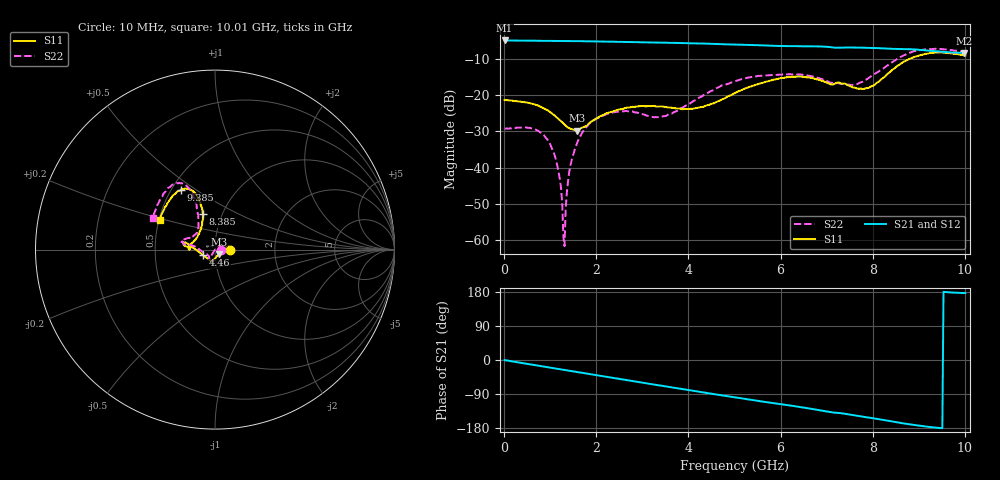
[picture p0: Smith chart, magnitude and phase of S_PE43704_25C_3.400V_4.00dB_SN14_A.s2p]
! Device ID: PE43704
! Dir: z:\PE43704\PE43704_Char_1_20130516\PE43704\AMB\3p400V\4p00dB
! Serial: 14
! Insertion: A
! Impedance: 50 ohm
! Temp: Amb
! VDD: 3.400V
! Attenuation Step: 4.00dB
! IDD: 1.140536e-01mA
#  Hz  S  RI  R  50
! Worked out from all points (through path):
!   401 points, 10 MHz to 10.01 GHz, reference 50 ohm
!   highest |S21| = -4.98 dB at 10 MHz (marker M1); lowest = -8.4 dB at 9.985 GHz (marker M2)
!   group delay of S21, straight-line fit = 52.4 ps
!   lowest |S11| = -29.9 dB at 1.585 GHz (marker M3), VSWR 1.07, Z = 52.1 - j2.5 ohm
!   |S11| at or under -10 dB: start of sweep to 8.807 GHz
!   |S22| runs from -61.7 to -7.3 dB; largest |S21 - S12| = 0.0043
!   S11 on the Smith chart (normalised r, x): 10 MHz: 1.19, +0.00; 4.46 GHz: 0.87, -0.06; 8.385 GHz: 0.81, +0.34; 9.385 GHz: 0.56, +0.44; 10.01 GHz: 0.50, +0.19
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1e7  0.085 0.000178  0.5634 -0.00236  0.5635 -0.00204  0.0343 0.000385
6.1e8  0.074 0.0163  0.5455 -0.1206  0.5453 -0.1205  0.0275 0.0209
9.35e8  0.0607 0.012  0.5263 -0.1807  0.5262 -0.1804  0.0172 0.0172
1.16e9  0.0479 0.00185  0.509 -0.2215  0.509 -0.2213  0.00672 0.00765
1.21e9  0.0449 -0.000908  0.5045 -0.2302  0.5047 -0.2301  0.00465 0.00504
1.26e9  0.0418 -0.0037  0.5001 -0.2391  0.5003 -0.2389  0.00192 0.00258
1.31e9  0.0385 -0.00692  0.4953 -0.2473  0.4955 -0.2473  -0.000311 -0.000766
1.435e9  0.0308 -0.0153  0.4832 -0.2681  0.4831 -0.268  -0.00603 -0.0085
1.585e9  0.0213 -0.024  0.4672 -0.2925  0.4673 -0.2923  -0.0116 -0.0185
1.685e9  0.0164 -0.0312  0.4559 -0.3083  0.4559 -0.308  -0.0159 -0.025
2.36e9  -0.0084 -0.0587  0.3661 -0.3985  0.3663 -0.3985  -0.0306 -0.0482
3.36e9  -0.0215 -0.0659  0.2068 -0.4838  0.2076 -0.4835  -0.0375 -0.032
4.46e9  -0.0666 -0.0316  0.0159 -0.5078  0.0163 -0.5081  -0.1096 0.0167
5.01e9  -0.1059 -0.000792  -0.0734 -0.4889  -0.0731 -0.4893  -0.1526 0.0247
6.685e9  -0.1696 0.022  -0.2961 -0.362  -0.2965 -0.3614  -0.1707 0.0573
7.585e9  -0.1175 0.0461  -0.3724 -0.2537  -0.3719 -0.2534  -0.099 0.0978
7.96e9  -0.086 0.099  -0.3965 -0.2023  -0.3963 -0.2036  -0.0924 0.1546
8.36e9  -0.0679 0.1924  -0.41 -0.1419  -0.4094 -0.1438  -0.1021 0.2447
8.385e9  -0.0676 0.1998  -0.411 -0.1377  -0.409 -0.1403  -0.103 0.2523
9.385e9  -0.1913 0.3328  -0.3986 -0.00988  -0.3993 -0.00807  -0.2462 0.3532
9.985e9  -0.3035 0.1763  -0.3788 0.0224  -0.3799 0.0234  -0.3407 0.1852
1.001e10  -0.3092 0.1651  -0.38 0.0226  -0.3818 0.0229  -0.3441 0.1765
